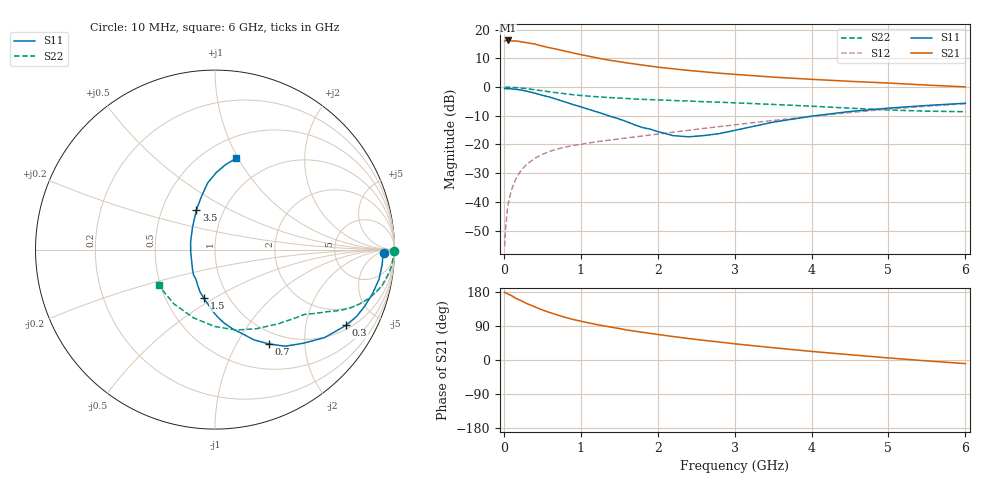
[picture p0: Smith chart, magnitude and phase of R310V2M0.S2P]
! SIEMENS Small Signal Semiconductors
! BFR181
! Si NPN RF Bipolar Junction Transistor in SOT23
! VCE = 10 V  IC = 2 mA
! Common Emitter S-Parameters:  May  1996
# GHz  S  MA  R  50
!  f  S11  S21  S12  S22
! GHz  MAG  ANG  MAG  ANG  MAG  ANG  MAG  ANG
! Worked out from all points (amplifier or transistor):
!   36 points, 10 MHz to 6 GHz, reference 50 ohm
!   highest |S21| = 16.2 dB at 50 MHz (marker M1)
!   |S21| within 3 dB of that: start of sweep to 679.6 MHz
!   unconditionally stable (mu >= 1): 1.678 GHz to 3.509 GHz
!   at 250 MHz: K = 0.23, MSG = 21.9 dB, |S12| = -28.3 dB
!   at 1.4 GHz: K = 0.92, MSG = 13.8 dB, |S12| = -18.4 dB
!   at 6 GHz: K = 0.86, MSG = 2.9 dB, |S12| = -5.8 dB
!   S11 on the Smith chart (normalised r, x): 10 MHz: 29, -10; 300 MHz: 1.15, -3.37; 700 MHz: 0.83, -1.37; 1.5 GHz: 0.77, -0.45; 3.5 GHz: 0.74, +0.35; 6 GHz: 0.70, +0.98
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0.01  0.9392 -1.2  6.362 178.6  0.0017 90.3  0.9968 -0.5
0.02  0.936 -2.0  6.362 177.4  0.0031 89.1  0.9853 -1.0
0.05  0.9351 -5.1  6.455 174.6  0.0085 86.3  0.9934 -2.6
0.1  0.9288 -10.2  6.325 169.8  0.0163 83.1  0.9885 -5.1
0.15  0.9112 -15.7  6.321 163.5  0.0243 79.5  0.9777 -7.6
0.2  0.8925 -20.5  6.224 158.7  0.0318 77.6  0.9642 -9.9
0.3  0.8436 -30.0  5.892 148.9  0.0456 72.3  0.9351 -14.0
0.4  0.7828 -38.8  5.605 140.5  0.0571 67.5  0.8967 -17.8
0.5  0.7177 -46.6  5.15 132.0  0.0671 63.8  0.859 -20.7
0.7  0.6039 -60.4  4.512 118.5  0.0835 58.7  0.7914 -25.0
0.8  0.5472 -66.7  4.192 112.4  0.0901 56.9  0.7625 -26.5
0.9  0.4945 -71.8  3.912 106.9  0.096 55.7  0.7348 -27.9
1.1  0.4101 -83.3  3.443 98.1  0.106 54.3  0.6937 -30.3
1.3  0.338 -92.9  3.044 90.1  0.1161 53.6  0.6643 -32.1
1.5  0.2778 -103.0  2.762 83.1  0.1252 53.8  0.6399 -34.0
1.7  0.2195 -116.3  2.517 76.1  0.1351 54.4  0.6179 -35.7
2.2  0.1427 -156.3  2.072 61.9  0.1636 55.2  0.5828 -41.2
2.8  0.1545 147.8  1.741 47.5  0.2047 54.9  0.5449 -49.3
3.5  0.2444 115.0  1.487 32.4  0.2616 52.4  0.4975 -62.4
4.5  0.375 96.1  1.255 13.9  0.3593 44.9  0.4283 -90.4
5.5  0.477 82.9  1.08 -2.4  0.4638 33.2  0.3794 -127.2
6  0.5217 77.0  1.005 -9.5  0.5128 26.1  0.3718 -147.5
